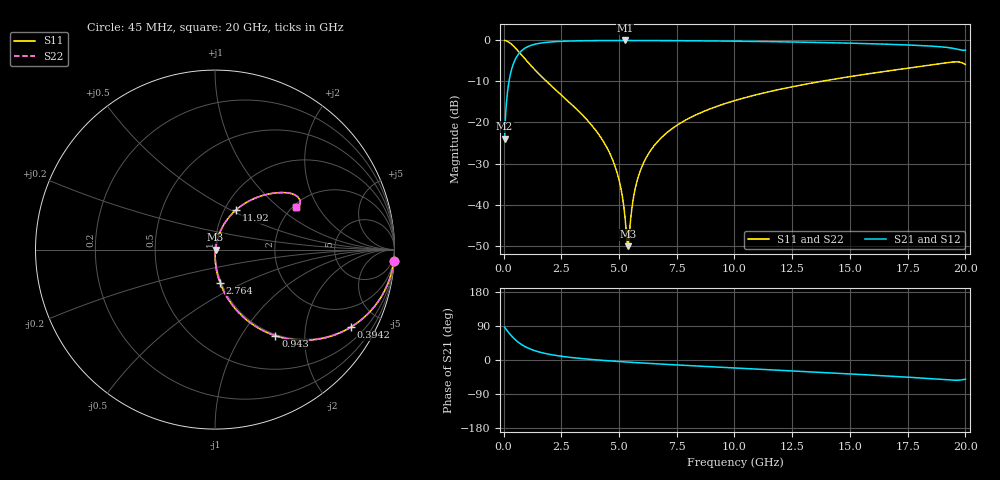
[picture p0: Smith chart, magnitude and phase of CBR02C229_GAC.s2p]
! S-parameter model data by Modelithics Inc.  support@modelithics.com 813-866-6335  Tampa FL USA
! S-Parameter data specifications:
! Substrate: 20-mil Rogers 4350B, substrate thickness, H=0.508mm, Dielectric constant, Er=3.75
! PCB Mounting Pad Footprint: Pad width, PadW=0.32mm , Pad length, PadL=0.37mm , Pad gap, PadG (edge-to-edge)=0.19mm , Reference planes=0.93mm apart
#  GHz  S  MA  R 50
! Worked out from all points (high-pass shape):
!   801 points, 45 MHz to 20 GHz, reference 50 ohm
!   highest |S21| = -0.03 dB at 5.258 GHz (marker M1); lowest = -23.9 dB at 45 MHz (marker M2)
!   |S21| within 3 dB of the highest: 691.6 MHz to end of sweep
!   lowest |S11| = -50.1 dB at 5.383 GHz (marker M3), VSWR 1.01, Z = 50.3 - j0.0385 ohm
!   |S11| at or under -10 dB: 1.863 GHz to 13.74 GHz (11.88 GHz wide, 152 % of centre)
!   |S22| runs from -50.1 to 0.0 dB; largest |S21 - S12| = 0
!   S11 on the Smith chart (normalised r, x): 45 MHz: 1, -31; 394.2 MHz: 0.98, -3.51; 943 MHz: 0.98, -1.43; 2.764 GHz: 0.99, -0.37; 11.92 GHz: 1.13, +0.54; 20 GHz: 2.09, +1.33
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0.045  0.998 -3.7  0.06373 86.3  0.06373 86.3  0.998 -3.7
0.219606  0.9545 -17.6  0.2979 72.4  0.2979 72.4  0.9545 -17.6
0.394213  0.8714 -29.7  0.49 60.2  0.49 60.2  0.8714 -29.7
0.942975  0.5864 -55.0  0.8088 34.9  0.8088 34.9  0.5864 -55.0
1.6414  0.3631 -70.1  0.93 19.6  0.93 19.6  0.3631 -70.1
2.763869  0.1854 -81.5  0.9804 7.8  0.9804 7.8  0.1854 -81.5
3.387462  0.1257 -85.2  0.9895 3.7  0.9895 3.7  0.1257 -85.2
4.185663  0.06738 -88.1  0.9949 -0.5  0.9949 -0.5  0.06738 -88.1
4.709481  0.03585 -88.2  0.9964 -2.8  0.9964 -2.8  0.03585 -88.2
5.03375  0.01824 -84.7  0.9967 -4.2  0.9967 -4.2  0.01824 -84.7
5.258244  0.007055 -69.2  0.9968 -5.1  0.9968 -5.1  0.007055 -69.2
5.382962  0.003117 -7.0  0.9968 -5.6  0.9968 -5.6  0.003117 -7.0
5.457794  0.004789 43.2  0.9968 -5.8  0.9968 -5.8  0.004789 43.2
5.657344  0.01364 69.8  0.9966 -6.6  0.9966 -6.6  0.01364 69.8
5.856894  0.02286 74.5  0.9964 -7.4  0.9964 -7.4  0.02286 74.5
6.704981  0.05997 76.3  0.9946 -10.4  0.9946 -10.4  0.05997 76.3
8.002056  0.1115 73.3  0.9897 -14.7  0.9897 -14.7  0.1115 73.3
10.0225  0.1852 67.6  0.978 -21.0  0.978 -21.0  0.1852 67.6
11.91822  0.2519 61.9  0.9623 -26.9  0.9623 -26.9  0.2519 61.9
13.36496  0.3029 57.5  0.9469 -31.4  0.9469 -31.4  0.3029 57.5
16.68248  0.4256 46.5  0.8965 -42.4  0.8965 -42.4  0.4256 46.5
20  0.5106 27.4  0.7605 -50.7  0.7605 -50.7  0.5106 27.4
